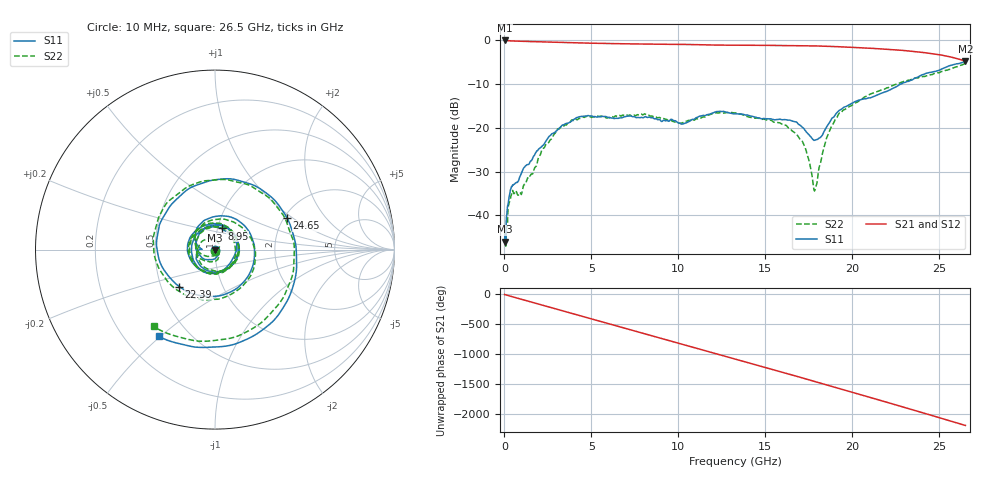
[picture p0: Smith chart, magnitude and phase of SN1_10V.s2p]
!Agilent Technologies,N5222A,MY51421700,A.10.00.00
!Agilent N5222A: A.10.00.00
!Date: Thursday, April 02, 2015 22:38:23
!Correction: S11(Full 2 Port(1,2))
!S21(Full 2 Port(1,2))
!S12(Full 2 Port(1,2))
!S22(Full 2 Port(1,2))
!S2P File: Measurements: S11, S21, S12, S22:
# Hz S  dB  R 50
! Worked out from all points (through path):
!   801 points, 10 MHz to 26.5 GHz, reference 50 ohm
!   highest |S21| = 0.01 dB at 10 MHz (marker M1); lowest = -4.7 dB at 26.5 GHz (marker M2)
!   group delay of S21, straight-line fit = 228 ps
!   lowest |S11| = -46.1 dB at 10 MHz (marker M3), VSWR 1.01, Z = 49.7 - j0.424 ohm
!   |S11| at or under -10 dB: start of sweep to 22.76 GHz
!   |S22| runs from -47.1 to -5.2 dB; largest |S21 - S12| = 0.0023
!   S11 on the Smith chart (normalised r, x): 10 MHz: 0.99, -0.01; 8.95 GHz: 1.05, +0.25; 22.39 GHz: 0.62, -0.28; 24.65 GHz: 2.07, +0.91; 26.5 GHz: 0.34, -0.49
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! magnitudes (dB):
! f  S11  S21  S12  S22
! 10 MHz  -46.1  0.0  0.0  -43.2
! 241.8 MHz  -36.5  -0.1  -0.1  -37.6
! 374.2 MHz  -33.9  -0.1  -0.1  -35.6
! 1.136 GHz  -29.1  -0.2  -0.2  -32.9
! 2.262 GHz  -23.8  -0.3  -0.3  -24.6
! 2.99 GHz  -20.7  -0.4  -0.4  -20.7
! 4.447 GHz  -17.4  -0.6  -0.6  -17.7
! 8.851 GHz  -18.1  -0.8  -0.8  -17.7
! 8.95 GHz  -18.2  -0.9  -0.9  -17.7
! 10.11 GHz  -19.0  -0.9  -0.9  -18.9
! 12.26 GHz  -16.3  -1.1  -1.1  -16.6
! 13.26 GHz  -16.8  -1.1  -1.1  -16.6
! 16.67 GHz  -18.6  -1.2  -1.2  -21.0
! 17.23 GHz  -20.3  -1.2  -1.2  -24.0
! 17.69 GHz  -22.4  -1.2  -1.2  -31.2
! 17.89 GHz  -22.8  -1.2  -1.2  -33.6
! 18.52 GHz  -19.8  -1.3  -1.3  -22.3
! 19.18 GHz  -16.3  -1.4  -1.4  -17.1
! 22.1 GHz  -11.4  -2.0  -2.0  -10.7
! 22.39 GHz  -10.9  -2.1  -2.1  -10.2
! 24.65 GHz  -7.2  -3.0  -3.0  -7.7
! 26.5 GHz  -4.8  -4.7  -4.7  -5.2
